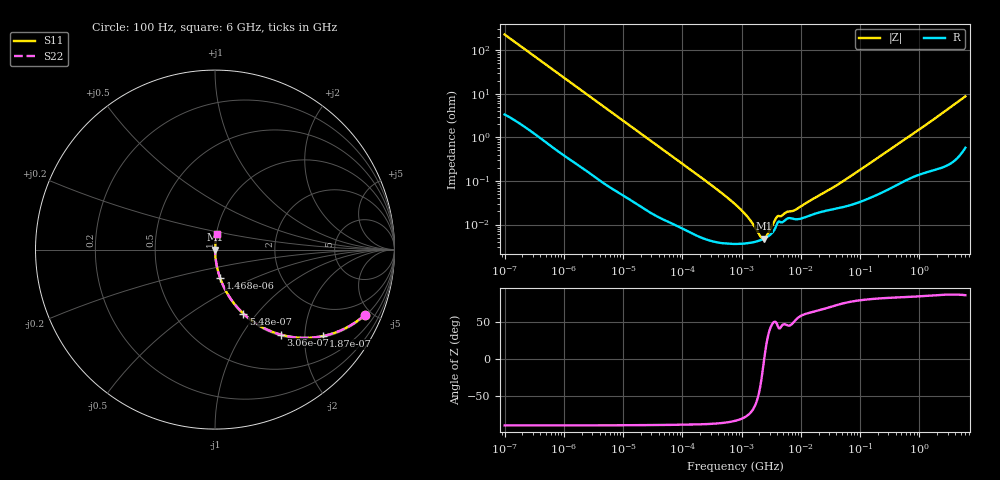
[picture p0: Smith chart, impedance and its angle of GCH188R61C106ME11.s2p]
!Murata Part Number: GCH188R61C106ME11
!These Parameters are Measured in Series Mode Connection
!Data Generated on Mar 13, 2026
!  o--ll--o
!Port1  Port2
!  o------o
!Operation Temp=25[degC], DC Bias Voltage=0[V]
!Freq. Start=100[Hz] Stop=6[GHz] 401[Steps]
# Hz S RI R 50
!Freq.(Hz) S11(Real) S11(Imag) S21(Real) S21(Imag) S12(Real) S12(Imag) S22(Real) S22(Imag)
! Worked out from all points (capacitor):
!   401 points, 100 Hz to 6 GHz, reference 50 ohm
!   read as one part in series: C = 6.91 uF near 109 Hz
!   lowest |Z| = 4.71 mohm at 2.373 MHz (marker M1)
!   series resonance near 2.408 MHz, so ESL is about 630 pH
!   S11 on the Smith chart (normalised r, x): 100 Hz: 1.07, -4.59; 187 Hz: 1.04, -2.47; 306 Hz: 1.03, -1.52; 548 Hz: 1.01, -0.85; 1.468 kHz: 1.01, -0.32; 6 GHz: 1.01, +0.17
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100  0.8368 -0.3623  0.1632 0.3623  0.1632 0.3623  0.8368 -0.3623
187  0.6024 -0.4814  0.3976 0.4814  0.3976 0.4814  0.6024 -0.4814
306  0.3677 -0.4739  0.6323 0.4739  0.6323 0.4739  0.3677 -0.4739
548  0.1582 -0.3568  0.8418 0.3568  0.8418 0.3568  0.1582 -0.3568
858  0.0734 -0.2527  0.9266 0.2527  0.9266 0.2527  0.0734 -0.2527
1468  0.0278 -0.1561  0.9722 0.1561  0.9722 0.1561  0.0278 -0.1561
2008  0.0157 -0.116  0.9843 0.116  0.9843 0.116  0.0157 -0.116
6433  0.00206 -0.0372  0.9979 0.0372  0.9979 0.0372  0.00206 -0.0372
40335  0.000183 -0.00607  0.9998 0.00607  0.9998 0.00607  0.000183 -0.00607
302498  4.28e-05 -0.000819  1 0.000819  1 0.000819  4.28e-05 -0.000819
774597  3.6e-05 -0.000293  1 0.000293  1 0.000293  3.6e-05 -0.000293
1585629  3.93e-05 -9.07e-05  1 9.07e-05  1 9.07e-05  3.93e-05 -9.07e-05
2372521  4.7e-05 -3.1e-06  1 3.1e-06  1 3.1e-06  4.7e-05 -3.1e-06
3245845  6.33e-05 6.71e-05  0.9999 -6.71e-05  0.9999 -6.71e-05  6.33e-05 6.71e-05
4060267  0.00011 0.000111  0.9999 -0.000111  0.9999 -0.000111  0.00011 0.000111
5809218  0.000135 0.00014  0.9999 -0.00014  0.9999 -0.00014  0.000135 0.00014
8311524  0.000132 0.000178  0.9999 -0.000178  0.9999 -0.000178  0.000132 0.000178
1.555665e7  0.000169 0.000337  0.9998 -0.000337  0.9998 -0.000337  0.000169 0.000337
4.764863e7  0.000246 0.000885  0.9998 -0.000885  0.9998 -0.000885  0.000246 0.000885
3.124326e8  0.000681 0.00511  0.9993 -0.00511  0.9993 -0.00511  0.000681 0.00511
1.873145e9  0.00256 0.0275  0.9974 -0.0275  0.9974 -0.0275  0.00256 0.0275
6e9  0.0131 0.0855  0.9869 -0.0855  0.9869 -0.0855  0.0131 0.0855
